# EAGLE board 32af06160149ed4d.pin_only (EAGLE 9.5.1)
REV: C

Size 25.4 x 17.78 mm. Coordinates in mm from the lower left corner, seen from the top.
Outline: 0,15.24 0,2.54 arc90 2.54,0 22.86,0 arc90 25.4,2.54 25.4,15.24 arc90 22.86,17.78 2.54,17.78 arc90 0,15.24
Copper layers (1*16): Top 0.035mm / dielectric 1.5mm / Bottom 0.035mm
Design rules "adafruit *": minimum track width 8mil, minimum drill 15.5mil, track to track 8mil, track to pad 8mil, pad to pad 8mil, via to via 8mil, smd to smd 8mil, copper to edge 10mil, drill to drill 8mil, minimum pad ring 10mil, minimum via ring 8mil, stop-mask expansion 2mil, vias tented up to drill 20mil, thermal gap 10mil
Net classes: 1 highpower: width 0.406 mm, drill 0.483 mm; 2 lowpower: width 0.305 mm, drill 0.483 mm

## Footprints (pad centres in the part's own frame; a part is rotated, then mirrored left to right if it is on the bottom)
0805-NO = smd 1.3 x 1.5: 1 -0.95,0; 2 0.95,0
0603-NO = smd 1.1 x 1: 1 -0.85,0; 2 0.85,0
JST_SH4 = smd 0.6 x 1.55: 1 -1.5,2.514; 2 -0.5,2.514; 3 0.5,2.514; 4 1.5,2.514 | smd 1.2 x 1.8: MT1 -2.8,-1.386; MT2 2.8,-1.386
SOD-323 = smd 1.35 x 0.8: A 1.27,0; C -1.27,0
CHIPLED_0603_NOOUTLINE = smd 0.8 x 0.8: A 0,-0.75; C 0,0.75
FIDUCIAL_1MM = smd 1 x 1: 1 0,0
1X06_ROUND_70 = drill 1 pad 1.778: 1 -6.35,0; 2 -3.81,0; 3 -1.27,0; 4 1.27,0; 5 3.81,0; 6 6.35,0
SOT363 = smd 0.5 x 0.5: 1 -0.75,-0.9; 3 0.75,-0.9; 4 0.75,0.9; 6 -0.75,0.9 | smd 0.4 x 0.5: 2 0,-0.9; 5 0,0.9
RESPACK_4X0603 = smd 0.45 x 0.9: 1 -1.3,-0.85; 2 -0.4,-0.85; 3 0.4,-0.85; 4 1.3,-0.85; 5 1.3,0.85; 6 0.4,0.85; 7 -0.4,0.85; 8 -1.3,0.85
VL6180 = smd 1 x 0.5: 1 -1.2,1.875; 2 -1.2,1.125; 3 -1.2,0.375; 4 -1.2,-0.375; 5 -1.2,-1.125; 6 -1.2,-1.875; 7 1.2,-1.875; 8 1.2,-1.125; 9 1.2,-0.375; 10 1.2,0.375; 11 1.2,1.125; 12 1.2,1.875
SOT23-5 = smd 0.55 x 1.2: 1 -0.95,-1.3; 2 0,-1.3; 3 0.95,-1.3; 4 0.95,1.3; 5 -0.95,1.3
MOUNTINGHOLE_2.5_PLATED = drill 2.5 pad 3.2: P$1 0,0

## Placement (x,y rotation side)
C4  10uF  [0805-NO]  7.62,5.59 0 top
C5  10uF  [0805-NO]  8.38,11.94 0 top
C6  0.1uF  [0603-NO]  10.16,8.51 270 top
CONN3  STEMMA_I2C_QT  [JST_SH4]  22.86,8.89 90 top
CONN4  STEMMA_I2C_QT  [JST_SH4]  2.54,8.89 270 top
D1  1N4148  [SOD-323]  17.14,5.84 180 top
D2  GREEN  [CHIPLED_0603_NOOUTLINE]  3.68,12.57 90 top
FID1  FIDUCIAL_1MM  [FIDUCIAL_1MM]  4.95,4.83 0 top
FID4  FIDUCIAL_1MM  [FIDUCIAL_1MM]  19.56,16.51 0 top
JP2  [1X06_ROUND_70]  12.7,2.54 0 top
Q3  BSS138  [SOT363]  17.53,8.64 90 top
R1  10K  [0603-NO]  12.7,12.32 180 top
R2  10K  [0603-NO]  12.7,5.59 180 top
R3  10K  [0603-NO]  5.84,12.45 90 top
R7  10K  [RESPACK_4X0603]  17.14,12.45 180 top
U1  VL6180X  [VL6180]  12.7,8.89 180 top
U3  LP5907-2.8V  [SOT23-5]  7.62,8.76 0 top
U$30  MOUNTINGHOLE2.5  [MOUNTINGHOLE_2.5_PLATED]  2.54,15.24 0 top
U$31  MOUNTINGHOLE2.5  [MOUNTINGHOLE_2.5_PLATED]  22.86,15.24 0 top
U$33  MOUNTINGHOLE2.5  [MOUNTINGHOLE_2.5_PLATED]  2.54,2.54 0 top
U$34  MOUNTINGHOLE2.5  [MOUNTINGHOLE_2.5_PLATED]  22.86,2.54 0 top
U$36  [ADAFRUIT_3.5MM]  4.57,13.72 0 top
U$37  [PCBFEAT-REV-040]  6.1,16.51 0 bottom
U$38  [STEMMAQT]  22.48,4.45 90 bottom
U$39  [STEMMAQT]  2.92,13.34 270 bottom

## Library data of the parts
C4-C6 CONN3 CONN4 D1 D2 JP2 Q3 R1-R3 R7 U1 U3 U$36 U$37 = microbuilder
FID1 FID4 U$30 U$31 U$33 U$34 = microbuilder; BOM: EXCLUDE
U$38 U$39 = silks

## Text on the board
tPlace: VL6180 | ToF Distance | on | GND | SDA | XSHUT | VIN | SCL | GPIO
bPlace: VL6180 | Time-of-Flight / Distance & Lux / Range: ~5-100mm | Vin/Vlogic: 3-5V

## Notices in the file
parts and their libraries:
microbuilder: This work is placed in the public domain, and may be freely used for commercial and non-commercial work with the following conditions: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
